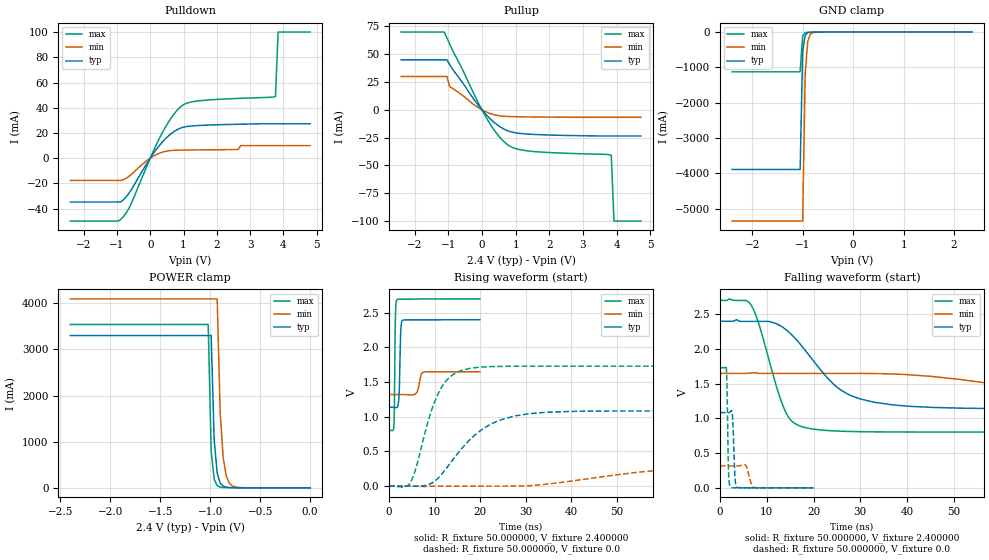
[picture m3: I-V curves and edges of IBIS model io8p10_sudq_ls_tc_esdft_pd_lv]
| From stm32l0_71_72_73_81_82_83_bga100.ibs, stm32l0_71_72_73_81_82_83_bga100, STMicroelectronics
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|   Model io8p10_sudq_ls_tc_esdft_pd_lv
[Model]  io8p10_sudq_ls_tc_esdft_pd_lv
Model_type I/O
Polarity   Non-Inverting
Enable   Active-Low
Vinl =   0.720000V
Vinh =   1.680000V
Vmeas =  1.200000V
Cref =   50.000000pF
Rref =   100.000000M
Vref =   0.0V
C_comp   2.242700pF   2.201100pF   2.288600pF
[Temperature Range]   25.000000   0.105000k   -40.000000
[Pullup Reference]   2.400000V   1.650000V   2.700000V
[Pulldown Reference]   0.0V   0.0V   0.0V
[POWER Clamp Reference]   2.400000V   1.650000V   2.700000V
[GND Clamp Reference]   0.0V   0.0V   0.0V
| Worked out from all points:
|   slope of the pulldown table from 0 to 0.36 V, typ, clamps not added: 28.4 ohm
|   slope of the pullup table from 0 to 0.36 V, typ, clamps not added: 32.2 ohm
|   GND clamp passes 1 mA (typ) near -0.64 V on its own axis
|   POWER clamp passes 1 mA (typ) near -0.63 V on its own axis
|   rising waveform, R_fixture 50.000000, V_fixture 2.400000: 20-80 % time 281ps typ, 635ps min, 186ps max; typ from 1.14 V to 2.4 V
|   rising waveform, R_fixture 50.000000, V_fixture 0.0: 20-80 % time 9.54ns typ, 25.2ns min, 4.93ns max; typ from 0 V to 1.08 V
|   falling waveform, R_fixture 50.000000, V_fixture 2.400000: 20-80 % time 10.1ns typ, 27.2ns min, 4.96ns max; typ from 2.4 V to 1.14 V
|   falling waveform, R_fixture 50.000000, V_fixture 0.0: 20-80 % time 354ps typ, 760ps min, 262ps max; typ from 1.08 V to 0 V
[Pulldown]
|Voltage   I(typ)   I(min)   I(max)
-2.4V     -34.71mA   -17.61mA   -49.77mA
-880mV    -34.55mA   -17.61mA   -48.41mA
-560mV    -24.66mA   -12.69mA   -35.31mA
240mV     8.893mA    3.542mA    13.9mA
560mV     17.98mA    5.931mA    29.16mA
880mV     23.58mA    6.389mA    40.03mA
1.44V     25.89mA    6.593mA    45.41mA
2.64V     26.92mA    7mA        47.38mA
2.72V     26.96mA    10mA       47.46mA
3.76V     27.3mA     10mA       49mA
3.84V     27.3mA     10mA       100mA
4.8V      27.3mA     10mA       100mA
[Pullup]
|Voltage   I(typ)   I(min)   I(max)
-2.4V     45mA       30mA       70mA
-1.12V    45mA       30mA       70mA
-1.04V    45mA       30mA       64.7mA
-960mV    40.7mA     21mA       59.3mA
80mV      -2.838mA   -1.261mA   -4.478mA
480mV     -14.04mA   -5.167mA   -22.91mA
800mV     -19.21mA   -5.978mA   -32.18mA
1.04V     -20.85mA   -6.184mA   -35.23mA
1.44V     -21.93mA   -6.373mA   -37.19mA
3.84V     -23.5mA    -6.7mA     -41mA
3.92V     -23.5mA    -6.7mA     -100mA
4.72V     -23.5mA    -6.7mA     -100mA
[GND_clamp]
|Voltage   I(typ)   I(min)   I(max)
-2.4V     -3.892A    -5.353A    -1.127A
-1.05V    -3.892A    -5.353A    -1.127A
-1V       -568.8mA   -5.353A    -105.4mA
-950mV    -88.96mA   -1.19A     -18.04mA
-900mV    -18.16mA   -269.2mA   -8.968mA
-850mV    -6.712mA   -63.46mA   -6.577mA
-800mV    -4.026mA   -16.62mA   -4.866mA
-650mV    -1.055mA   -1.234mA   -1.154mA
2.35V     53.38uA    50.3uA     37.53uA
[POWER_clamp]
|Voltage   I(typ)   I(min)   I(max)
-2.4V     3.303A     4.097A     3.542A
-1.02V    3.303A     4.097A     3.542A
-990mV    3.303A     4.097A     802.4mA
-960mV    1.032A     4.097A     186.5mA
-930mV    325.2mA    4.097A     47.59mA
-900mV    104.8mA    1.637A     15.78mA
-870mV    35.83mA    655.7mA    8.015mA
-840mV    13.93mA    263.9mA    5.668mA
-810mV    6.712mA    107.2mA    4.56mA
-780mV    4.088mA    44.39mA    3.763mA
-690mV    1.741mA    4.361mA    1.91mA
0V        0A         0A         0A
[Ramp]
| variable   typ   min   max
dV/dt_r  0.65004/9.52767n   0.18967/25.20006n   1.03746/4.90940n
dV/dt_f  0.75702/10.10896n   0.19728/27.24333n   1.13765/4.95734n
R_load = 50.000000
[Rising Waveform]
R_fixture= 50.000000
V_fixture= 2.400000
V_fixture_min= 1.650000
V_fixture_max= 2.700000
|time   V(typ)   V(min)   V(max)
0s        1.137V     1.32V      803.3mV
1.041ns   1.137V     1.32V      874.9mV
1.161ns   1.136V     1.32V      1.218V
1.361ns   1.133V     1.32V      2.398V
1.722ns   1.132V     1.32V      2.687V
2.122ns   1.254V     1.32V      2.695V
2.563ns   2.249V     1.32V      2.695V
2.963ns   2.391V     1.32V      2.696V
7.568ns   2.396V     1.642V     2.698V
19.94ns   2.399V     1.649V     2.699V
[Rising Waveform]
R_fixture= 50.000000
V_fixture= 0.0
V_fixture_min= 0.0
V_fixture_max= 0.0
|time   V(typ)   V(min)   V(max)
0s        -407.5nV   -2.921uV   -29.65nV
5.005ns   -681.5uV   102.7uV    92.86mV
9.51ns    47.92mV    -154.5uV   1.129V
12.01ns   209.7mV    -150.8uV   1.474V
15.02ns   466.3mV    -154.4uV   1.644V
20.02ns   797.4mV    -111.4uV   1.716V
27.53ns   1.01V      1.382mV    1.728V
42.04ns   1.08V      91.03mV    1.729V
90.09ns   1.083V     307.6mV    1.729V
249.2ns   1.083V     316.1mV    1.729V
[Falling Waveform]
R_fixture= 50.000000
V_fixture= 2.400000
V_fixture_min= 1.650000
V_fixture_max= 2.700000
|time   V(typ)   V(min)   V(max)
0s        2.399V     1.649V     2.699V
6.507ns   2.397V     1.654V     2.647V
8.008ns   2.397V     1.65V      2.421V
14.51ns   2.256V     1.647V     1.032V
21.52ns   1.697V     1.647V     833mV
25.53ns   1.423V     1.647V     816.6mV
30.03ns   1.279V     1.647V     808.9mV
45.55ns   1.158V     1.603V     803.6mV
96.6ns    1.137V     1.341V     803.3mV
249.2ns   1.137V     1.32V      803.3mV
[Falling Waveform]
R_fixture= 50.000000
V_fixture= 0.0
V_fixture_min= 0.0
V_fixture_max= 0.0
|time   V(typ)   V(min)   V(max)
0s        1.083V     316.1mV    1.729V
1.361ns   1.083V     316.1mV    1.718V
1.522ns   1.083V     316.1mV    1.369V
1.802ns   1.083V     316.1mV    286.8mV
2.202ns   1.096V     316.1mV    14.4mV
2.643ns   1.053V     316.1mV    1.462mV
3.203ns   151mV      315.9mV    992.9uV
3.644ns   7.991mV    315.6mV    1.009mV
7.287ns   333.5uV    5.618mV    1.155mV
19.94ns   -407.5nV   -2.921uV   -29.65nV
